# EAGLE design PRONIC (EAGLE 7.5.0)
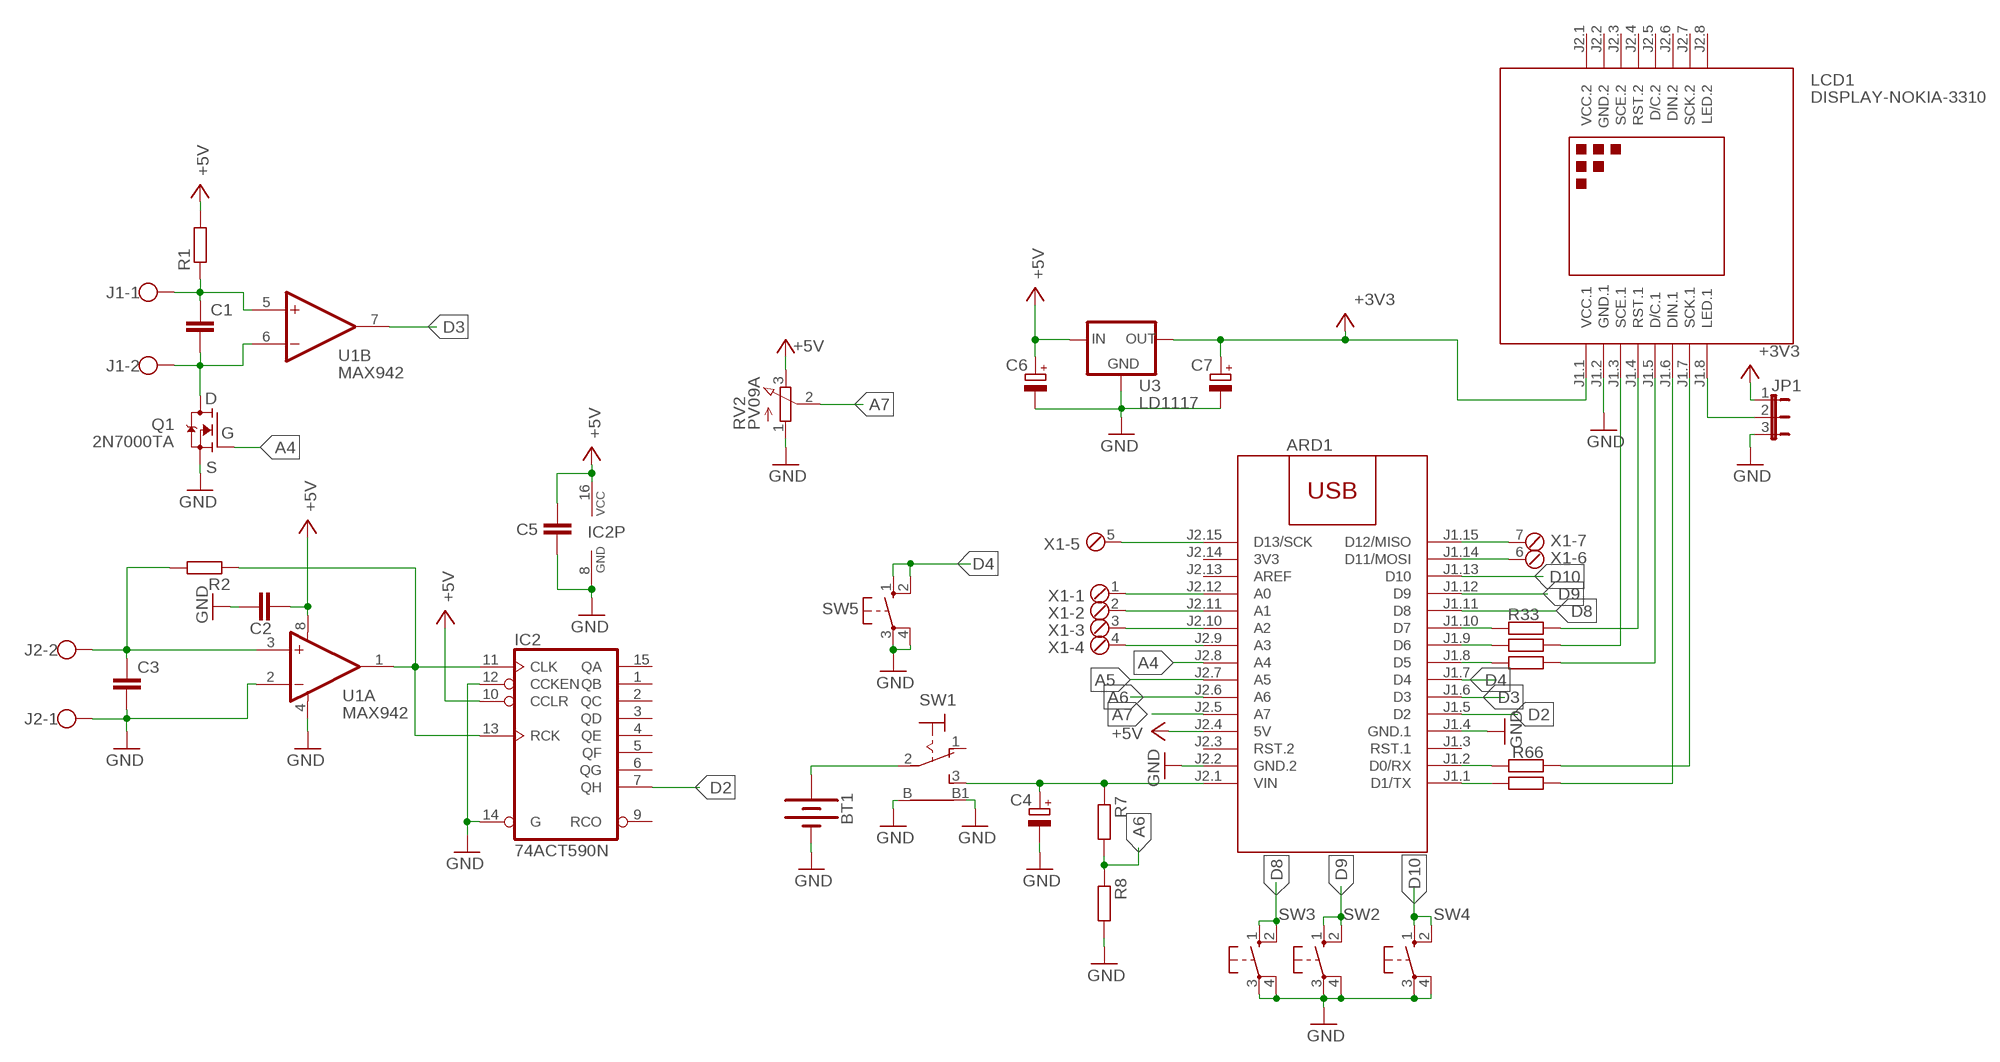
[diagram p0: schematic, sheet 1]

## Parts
ARD1  ARDUINO-NANO-3.0  [ARDUINO-NANO-3.0]
BT1  BATTERY-9V  [BATTCON_9V]
C1  C-EUC1206  [C1206]
C2  C-EUC1206  [C1206]
C3  C-EUC1206  [C1206]
C4  CPOL-EUSMCC  [SMC_C]
C5  C-EUC1206  [C1206]
C6  CPOL-EUSMCB  [SMC_B]
C7  CPOL-EUSMCB  [SMC_B]
IC2  74ACT590N  [DIL16]
J1  W237-102  [W237-102]
J2  W237-102  [W237-102]
JP1  JP2E  [JP2]
LCD1  DISPLAY-NOKIA-3310  [DISPLAY-NOKIA-3310]
Q1  2N7000TA  [TO-92]
R1  R-EU_R1206  [R1206]
R2  R-EU_R1206  [R1206]
R7  R-EU_R1206  [R1206]
R8  R-EU_R1206  [R1206]
R22  R-EU_R1206  [R1206]
R33  R-EU_R1206  [R1206]
R44  R-EU_R1206  [R1206]
R55  R-EU_R1206  [R1206]
R66  R-EU_R1206  [R1206]
RV2  PV09A  [PTV09]
SW1  9070-1W  [9070-1W]
SW2  40-XX  [B3F-40XX]
SW3  40-XX  [B3F-40XX]
SW4  40-XX  [B3F-40XX]
SW5  40-XX  [B3F-40XX]
U1  MAX942  MAX907CPA  [DIL08]
U3  LD1117  [SOT223]
X1  MPT7  [7POL254]

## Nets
+3V3: C7.+ JP1.1 LCD1.J1.1(VCC.1) U3.2(OUT)
+5V: ARD1.J2.4(5V) C2.2 C5.2 C6.+ IC2.10(CCLR) IC2.16(VCC) R1.2 RV2.3(E) U1.8(A:V+) U3.3(IN)
A4: ARD1.J2.8(A4) Q1.2(G)
A5: ARD1.J2.7(A5)
A6: ARD1.J2.6(A6) R7.2 R8.1
A7: ARD1.J2.5(A7) RV2.2(S)
D2: ARD1.J1.5(D2) IC2.7(QH)
D3: ARD1.J1.6(D3) U1.7(B:OUT)
D4: ARD1.J1.7(D4) SW5.1(S) SW5.2(S1)
D8: ARD1.J1.11(D8) SW3.1(S) SW3.2(S1)
D9: ARD1.J1.12(D9) SW2.1(S) SW2.2(S1)
D10: ARD1.J1.13(D10) SW4.1(S) SW4.2(S1)
GND: ARD1.J1.4(GND.1) ARD1.J2.2(GND.2) BT1.- C2.1 C3.2 C4.- C5.1 C6.- C7.- IC2.8(GND) IC2.12(CCKEN) IC2.14(G) J2.1 JP1.3 LCD1.J1.2(GND.1) Q1.1(S) R8.2 RV2.1(A) SW1.B SW1.B1 SW2.3(P) SW2.4(P1) SW3.3(P) SW3.4(P1) SW4.3(P) SW4.4(P1) SW5.3(P) SW5.4(P1) U1.2(A:-IN) U1.4(A:V-) U3.1(GND)
N$1: ARD1.J1.1(D1/TX) R55.2
N$2: LCD1.J1.6(DIN.1) R55.1
N$3: ARD1.J1.10(D7) R33.2
N$4: ARD1.J1.9(D6) R22.2
N$5: ARD1.J1.8(D5) R44.2
N$6: ARD1.J1.2(D0/RX) R66.2
N$7: ARD1.J2.12(A0) X1.1
N$8: LCD1.J1.4(RST.1) R33.1
N$9: LCD1.J1.3(SCE.1) R22.1
N$10: LCD1.J1.5(D/C.1) R44.1
N$11: ARD1.J2.11(A1) X1.2
N$12: LCD1.J1.7(SCK.1) R66.1
N$13: JP1.2 LCD1.J1.8(LED.1)
N$14: ARD1.J2.10(A2) X1.3
N$15: ARD1.J2.9(A3) X1.4
N$16: ARD1.J2.15(D13/SCK) X1.5
N$17: ARD1.J1.14(D11/MOSI) X1.6
N$18: ARD1.J1.15(D12/MISO) X1.7
N$19: C1.1 J1.1 R1.1 U1.5(B:+IN)
N$20: C1.2 J1.2 Q1.3(D) U1.6(B:-IN)
N$21: C3.1 J2.2 R2.2 U1.3(A:+IN)
N$22: IC2.11(CLK) IC2.13(RCK) R2.1 U1.1(A:OUT)
N$24: BT1.+ SW1.2(P)
N$25: ARD1.J2.1(VIN) C4.+ R7.1 SW1.3(S)
Unconnected: ARD1.J1.3(RST.1) ARD1.J2.3(RST.2) ARD1.J2.13(AREF) IC2.1(QB) IC2.2(QC) IC2.3(QD) IC2.4(QE) IC2.5(QF) IC2.6(QG) IC2.9(RCO) IC2.15(QA) LCD1.J2.3(SCE.2) LCD1.J2.4(RST.2) LCD1.J2.5(D/C.2) LCD1.J2.6(DIN.2) LCD1.J2.7(SCK.2) LCD1.J2.8(LED.2) SW1.1(O)

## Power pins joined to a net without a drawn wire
3V3: ARD1.J2.14(3V3)
GND.2: LCD1.J2.2(GND.2)
VCC.2: LCD1.J2.1(VCC.2)

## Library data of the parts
ARD1 = diy-modules:ARDUINO-NANO-3.0: Arduino Nano 3.0 and compatible devices More details available here: https://www.arduino.cc/en/Main/ArduinoBoardNano Click here to find device on ebay.com
BT1 = SparkFun-Batteries:BATTERY: Battery - Single Cell; PROD_ID: BATT-10855
C1-C3 C5 = rcl:C-EU: CAPACITOR, European symbol
C4 C6 C7 = rcl:CPOL-EU: POLARIZED CAPACITOR, European symbol
IC2 = 74xx-eu:74*590: 8-bit binary COUNTER, output register
J1 J2 = con-wago-500:W237-102: WAGO SCREW CLAMP; MPN: 237-102; OC_FARNELL: unknown; OC_NEWARK: 70K9898
JP1 = jumper:JP2E: JUMPER
LCD1 = diy-modules:DISPLAY-NOKIA-3310: 84x48 Dot Matrix LCD Module based on Nokia 3310 display More details available here: https://arduinoandsoftware.wordpress.com/2012/12/30/nokia-33105110-3-3v-display-with-5v-arduino/
Q1 = 2N7000TA:2N7000TA: http://www.mouser.com/ds/2/149/2N7000TA-347571.pdf Check availability; AVAILABILITY: In Stock; CHECK_PRICES: https://www.snapeda.com/parts/2N7000-TA/Onsemi/view-part/?ref=eda; DESCRIPTION: N-Channel 60 V 200mA (Tc) 400mW (Ta) Through Hole TO-92-3; MF: ON Semiconductor; MP: 2N7000-TA; PACKAGE: E-PKG AXIAL-LEADED-2 ON Semiconductor; PRICE: None; SNAPEDA_LINK: https://www.snapeda.com/parts/2N7000-TA/Onsemi/view-part/?ref=snap
R1 R2 R7 R8 R22 R33 R44 R55 R66 = rcl:R-EU_: RESISTOR, European symbol
RV2 = pot:PV09A
SW1 = switch:9070-1W: TOGGLE SWITCH Marquardt
SW2-SW5 = switch-omron:40-XX: OMRON SWITCH; MF: OMRON COMPONENTS USA; MPN: B3F-4000; OC_FARNELL: 176434; OC_NEWARK: 36K3105
U1 = maxim:MAX907CPA: COMPARATOR; MF: MAXIM; MPN: MAX907CPA; OC_FARNELL: unknown; OC_NEWARK: 79C3004
U3 = v-reg:LD1117
X1 = con-phoenix-254:MPT7: PHOENIX CONNECTOR; OC_FARNELL: unknown; OC_NEWARK: unknown

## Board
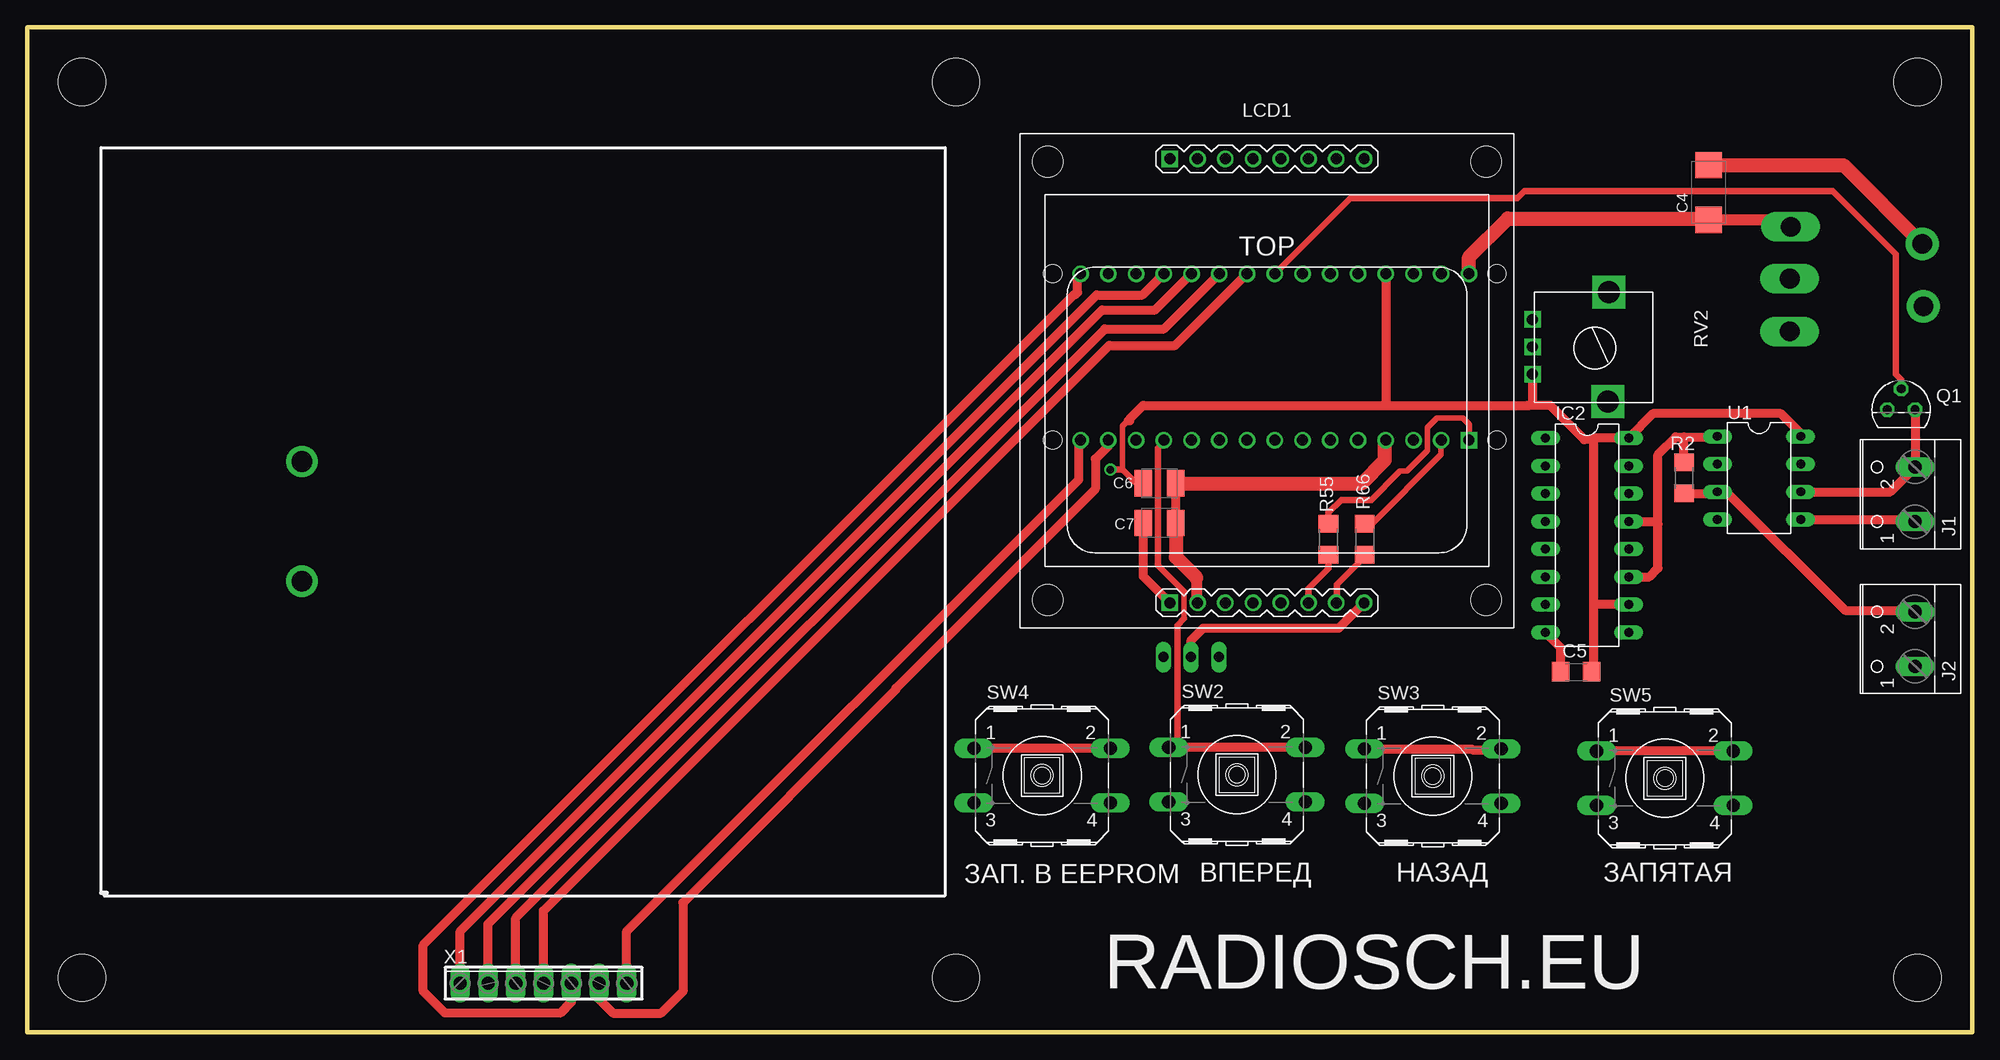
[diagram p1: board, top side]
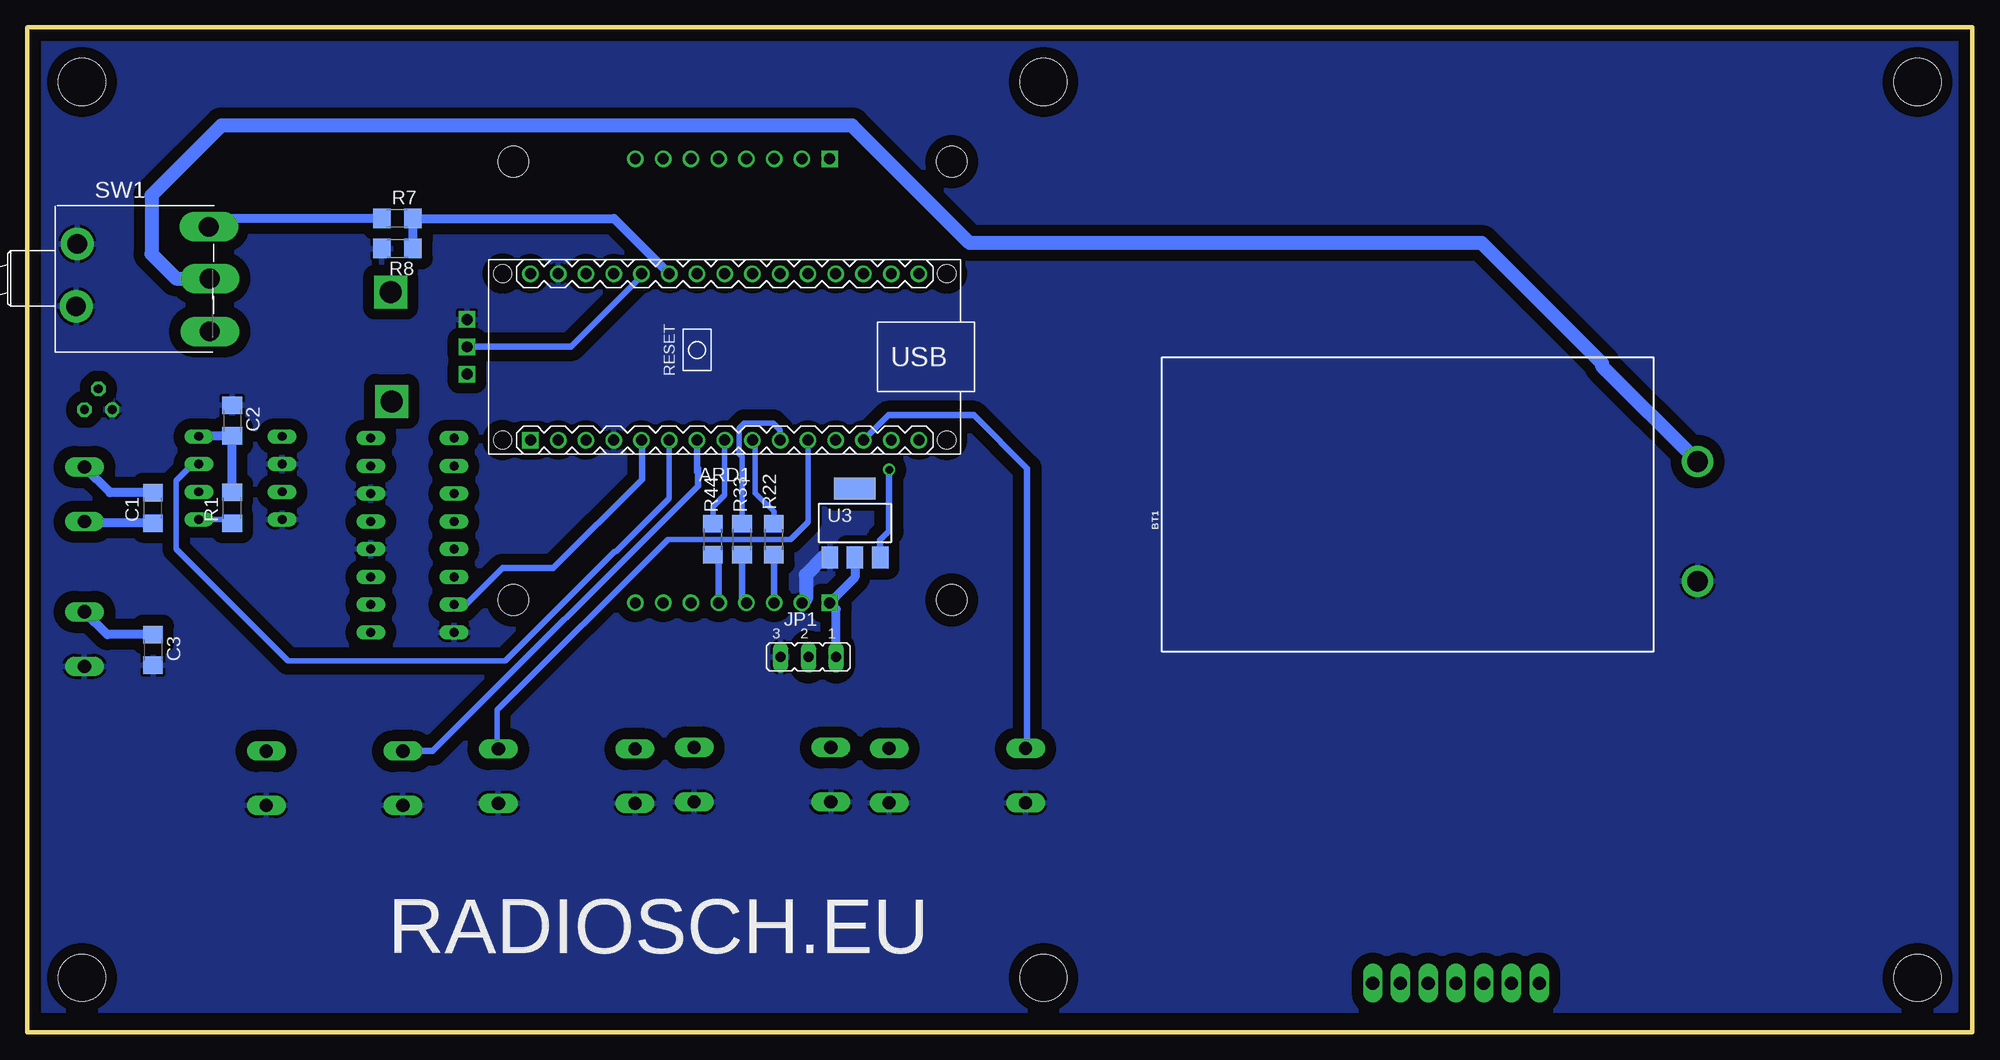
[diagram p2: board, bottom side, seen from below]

Size 178 x 92 mm. Coordinates in mm from the lower left corner, seen from the top.
Outline: 0,0 178,0 178,92 0,92 0,0
Copper layers (1*16): Top 0.035mm / dielectric 1.5mm / Bottom 0.035mm
Design rules "default": minimum track width 10mil, minimum drill 24mil, track to track 8mil, track to pad 8mil, pad to pad 8mil, via to via 8mil, smd to smd 8mil, copper to edge 40mil, drill to drill 8mil, minimum pad ring 10mil, minimum via ring 8mil, stop-mask expansion 4mil, vias tented up to drill 0mil, thermal gap 10mil
Holes 4.3 mm at 5,5 173,5 5,87 85,5 85,87 173,87

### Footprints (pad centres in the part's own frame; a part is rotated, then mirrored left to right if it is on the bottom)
ARDUINO-NANO-3.0 = drill 1 square: J1.1 17.78,7.62 | drill 1: J1.2 15.24,7.62; J1.3 12.7,7.62; J1.4 10.16,7.62; J1.5 7.62,7.62; J1.6 5.08,7.62; J1.7 2.54,7.62; J1.8 0,7.62; J1.9 -2.54,7.62; J1.10 -5.08,7.62; J1.11 -7.62,7.62; J1.12 -10.16,7.62; J1.13 -12.7,7.62; J1.14 -15.24,7.62; J1.15 -17.78,7.62; J2.1 17.78,-7.62; J2.2 15.24,-7.62; J2.3 12.7,-7.62; J2.4 10.16,-7.62; J2.5 7.62,-7.62; J2.6 5.08,-7.62; J2.7 2.54,-7.62; J2.8 0,-7.62; J2.9 -2.54,-7.62; J2.10 -5.08,-7.62; J2.11 -7.62,-7.62; J2.12 -10.16,-7.62; J2.13 -12.7,-7.62; J2.14 -15.24,-7.62; J2.15 -17.78,-7.62 | hole 1.651: -20.32,7.62; -20.32,-7.62; 20.32,-7.62; 20.32,7.62
BATTCON_9V = drill 1.905: + -4,-1; - -4,-11.954
C1206 = smd 1.6 x 1.8: 1 -1.4,0; 2 1.4,0
SMC_C = smd 2.4 x 2.4: + -2.5,0; - 2.5,0
SMC_B = smd 1.6 x 2.4: + -1.5,0; - 1.5,0
DIL16 = drill 0.813 long: 1 -8.89,-3.81; 2 -6.35,-3.81; 3 -3.81,-3.81; 4 -1.27,-3.81; 5 1.27,-3.81; 6 3.81,-3.81; 7 6.35,-3.81; 8 8.89,-3.81; 9 8.89,3.81; 10 6.35,3.81; 11 3.81,3.81; 12 1.27,3.81; 13 -1.27,3.81; 14 -3.81,3.81; 15 -6.35,3.81; 16 -8.89,3.81
W237-102 = drill 1.194 long: 1 -2.5,-1.27; 2 2.5,-1.27
JP2 = drill 0.914 long: 1 -2.54,0; 2 0,0; 3 2.54,0
DISPLAY-NOKIA-3310 = drill 1 square: J1.1 -8.89,-20.32; J2.1 -8.89,20.32 | drill 1: J1.2 -6.35,-20.32; J1.3 -3.81,-20.32; J1.4 -1.27,-20.32; J1.5 1.27,-20.32; J1.6 3.81,-20.32; J1.7 6.35,-20.32; J1.8 8.89,-20.32; J2.2 -6.35,20.32; J2.3 -3.81,20.32; J2.4 -1.27,20.32; J2.5 1.27,20.32; J2.6 3.81,20.32; J2.7 6.35,20.32; J2.8 8.89,20.32 | hole 2.8: -20.066,-20.066; 20.066,-20.066; 20.066,20.066; -20.066,20.066
TO-92 = drill 0.813 octagon: 1 -1.27,0; 2 0,1.905; 3 1.27,0
R1206 = smd 1.6 x 1.803: 1 -1.422,0; 2 1.422,0
PTV09 = drill 1 square: 1 -2.5,0; 2 0,0; 3 2.5,0 | drill 2 square: P$4 -5,7; P$5 5,6.9
9070-1W = drill 1.813 long: 1 5.08,-4.835; 2 5.08,0 | drill 1.8 long: 3 4.98,4.735 | drill 1.8 pad 3: B -7.161,-2.544; B1 -7.061,3.167
B3F-40XX = drill 1.194 long: 1 -6.248,2.489; 2 6.248,2.489; 3 -6.248,-2.489; 4 6.248,-2.489
DIL08 = drill 0.813 long: 1 -3.81,-3.81; 2 -1.27,-3.81; 3 1.27,-3.81; 4 3.81,-3.81; 5 3.81,3.81; 6 1.27,3.81; 7 -1.27,3.81; 8 -3.81,3.81
SOT223 = smd 1.5 x 2: 1 -2.3,-3.15; 2 0,-3.15; 3 2.3,-3.15 | smd 3.8 x 2: 4 0,3.15
7POL254 = drill 1.2 long: 1 -7.62,0; 2 -5.08,0; 3 -2.54,0; 4 0,0; 5 2.54,0; 6 5.08,0; 7 7.62,0

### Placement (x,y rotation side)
ARD1  114.17,61.83 180 bottom
BT1  21.12,53.25 0 bottom
C1  166.5,48 90 bottom
C2  159.25,56 270 bottom
C3  166.5,35 270 bottom
C4  153.88,76.88 90 top
C5  141.75,33 0 top
C6  103.62,50.25 0 top
C7  103.62,46.62 0 top
IC2  142.75,45.5 270 top
J1  171.5,49.25 90 top
J2  171.5,36 90 top
JP1  106.51,34.35 180 bottom
LCD1  113.46,59.64 0 top
Q1  171.5,57 0 top
R1  159.25,48 90 bottom
R2  151.62,50.75 270 top
R7  144.12,74.5 0 bottom
R8  144.12,71.75 180 bottom
R22  109.67,45.13 90 bottom
R33  112.59,45.13 90 bottom
R44  115.25,45.13 90 bottom
R55  119.08,45.13 90 top
R66  122.41,45.13 90 top
RV2  137.75,62.75 270 top
SW1  166.38,69 0 bottom
SW2  110.71,23.58 0 top
SW3  128.64,23.45 0 top
SW4  92.88,23.5 0 top
SW5  149.88,23.25 0 top
U1  158.5,50.75 270 top
U3  102.25,46.62 0 bottom
X1  47.25,4.5 0 top

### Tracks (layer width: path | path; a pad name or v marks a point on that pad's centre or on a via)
+3V3
  Top 0.813: C7.+ 102.12,41.77 LCD1.J1.1
  Bottom 0.813: JP1.1 103.97,38.72 LCD1.J1.1 102.25,41.64 U3.2
+5V  (via drill 0.7)
  Top 0.5: C6.+ 101.5,50.25 100.25,51.5 100.25,55.5 100.75,56
  Top 0.61: v99.12,51.5 100.25,51.5
  Top 0.813: 100.75,56 100.88,56 100.88,56.12 102.12,57.38 124.62,57.38 | 124.62,57.38 137.25,57.38 137.5,57.38 | 143.38,39 143.38,33.23 C5.2 | 143.38,39 143.38,54.25 | 143.38,54.25 143.51,54.39 IC2.16 148.79,56.62 160.5,56.62 162.31,54.81 U1.8 | ARD1.J2.4 124.33,57.67 124.62,57.38 | IC2.10 143.53,39.15 143.38,39 | RV2.3 137.75,57.62 137.5,57.38 | 143.38,54.25 142.5,54.25 139.38,57.38 137.5,57.38
  Bottom 0.61: U3.3 99.95,45.05 99.12,45.88 v99.12,51.5
  Bottom 0.813: R1.2 C2.2 162.27,54.6 U1.8
A4
  Top 0.61: ARD1.J2.8 121.09,76.38 136.38,76.38 137,77 165.25,77 171,71.25 171,60.25 171.5,59.75 Q1.2
A6
  Bottom 0.813: ARD1.J2.6 124.3,74.5 R7.2 R8.1
A7
  Bottom 0.61: RV2.2 128.25,62.75 122.12,68.88 122.12,69.11 ARD1.J2.5
D2
  Bottom 0.61: IC2.7 137.85,39.15 134.5,42.5 129.88,42.5 121.75,50.62 121.75,54.17 ARD1.J1.5
D3
  Bottom 0.5: ARD1.J1.6 119.25,48.88 124.12,44 124.25,44 134.25,34 154.12,34 164.38,44.25 164.38,50.5 162.88,52 162.33,52 U1.7
D4
  Top 0.813: SW5.2 SW5.1
  Bottom 0.61: ARD1.J1.7 116.71,51.75 | 116.71,51.75 116.71,51.29 | SW5.1 140.89,25.74 116.62,50 116.62,51.66 116.71,51.75
D8
  Top 0.813: 122.41,25.95 SW3.1 132.19,25.94 132.25,25.88 134.82,25.88 SW3.2
  Bottom 0.5: ARD1.J1.11 106.55,46.7 108.12,45.12 119.38,45.12 135,29.5 135,26.05 SW3.2
D9
  Top 0.5: 105.88,40.38 105.88,37.88
  Top 0.61: ARD1.J1.12 104.01,54.01 103.5,53.5 103.5,42.75 105.88,40.38 | 105.88,37.88 105.25,37.25 105.25,26.86 SW2.1
  Top 0.813: SW2.2 SW2.1
D10
  Top 0.813: SW4.2 SW4.1
  Bottom 0.61: SW4.1 86.5,26.12 86.5,51.62 91.38,56.5 99.18,56.5 ARD1.J1.13
GND
  Top 0.813: C7.- C6.- | C5.1 140.35,35.2 IC2.8
  Top 1.016: 107,41.62 107,39.43
  Top 1.27: C6.- 122.12,50.25 124.25,52.38 124.25,54.13 ARD1.J1.4 | C7.- 105.12,43.5 107,41.62 | 107,39.43 LCD1.J1.2 | C4.- 166.23,79.38 SW1.B1
  Bottom 1.27: U3.1 105.15,43.48 106.75,41.88 106.75,39.68 LCD1.J1.2
  pour Bottom (isolate 1.016): 1.5,2 177,2 177,91 1.5,91
N$1
  Top 0.5: 125.5,51.25 125.62,51.38 126.25,51.38 128.12,53.25 128.12,55.38 129,56.25 131.38,56.25 132,55.62 132,54.26 ARD1.J1.1
  Top 0.61: R55.2 119.08,47.58 120.25,48.75 123,48.75 125.5,51.25
N$2
  Top 0.61: R55.1 119.08,42.45 117.25,40.62 117.25,39.34 LCD1.J1.6
N$3
  Bottom 0.5: R33.2 112.59,52.72 112.88,53 112.88,55.25 112.38,55.75 109.75,55.75 109.12,55.12 109.12,54.24 ARD1.J1.10
N$4
  Bottom 0.5: R22.2 109.67,47.67 111.38,49.38 111.38,53.95 ARD1.J1.9
N$5
  Bottom 0.5: ARD1.J1.8 114.17,49.2 115.25,48.12 R44.2
N$6
  Top 0.5: R66.2 123.05,46.55 129.38,52.88 129.38,54.17 ARD1.J1.2
N$7
  Top 0.813: X1.1 39.63,9.26 97.88,67.5 102.06,67.5 ARD1.J2.12
N$8
  Bottom 0.61: R33.1 112.59,39.72 LCD1.J1.4
N$9
  Bottom 0.61: R22.1 109.67,39.34 LCD1.J1.3
N$10
  Bottom 0.61: LCD1.J1.5 114.73,43.19 R44.1
N$11
  Top 0.813: X1.2 42.17,9.92 98.38,66.12 103.22,66.12 ARD1.J2.11
N$12
  Top 0.61: R66.1 122.41,43.53 119.88,41 119.88,39.38 LCD1.J1.7
N$13
  Top 0.813: JP1.2 106.51,35.88 107.62,37 120.03,37 LCD1.J1.8
N$14
  Top 0.813: X1.3 44.71,10.46 98.62,64.38 104.02,64.38 ARD1.J2.10
N$15
  Top 0.813: X1.4 47.25,11.12 99,62.88 105.06,62.88 ARD1.J2.9
N$16
  Top 0.813: X1.5 49.79,2.79 48.75,1.75 38.25,1.75 36.25,3.75 36.25,8 95.75,67.5 95.88,67.5 96.12,67.75 96.12,69.19 ARD1.J2.15
N$17
  Top 0.813: ARD1.J1.14 98.93,53.68 97.75,52.5 97.75,49.75 79.5,31.5 79.5,31.38 60,11.88 60,3.75 58,1.75 53.62,1.75 52.25,3.12 52.25,4.42 X1.6
N$18
  Top 0.813: X1.7 54.87,9.24 96.25,50.62 96.25,54.07 ARD1.J1.15
N$19
  Top 0.813: U1.5 172.58,46.94 J1.1
  Bottom 0.5: U1.5 159.61,46.94 R1.1
  Bottom 0.813: C1.1 172.62,46.6 J1.1
N$20
  Top 0.813: U1.6 170.5,49.48 J1.2 Q1.3
  Bottom 0.813: C1.2 170.42,49.4 J1.2
N$21
  Top 0.813: R2.2 154.54,49.33 U1.3 155.52,49.48 166.38,38.62 172.65,38.62 J2.2
  Bottom 0.813: C3.1 170.67,36.4 J2.2
N$22
  Top 0.813: IC2.11 148.44,41.69 149.25,42.5 149.25,46.5 | 149.25,46.5 149.25,52.88 150.88,54.5 151.62,54.5 | 151.62,54.5 154.63,54.5 U1.1 | R2.1 151.62,54.5 | IC2.13 148.98,46.77 149.25,46.5
N$24
  Bottom 1.27: BT1.+ 33.88,61 33.88,61.25 44.88,72.25 91.75,72.25 102.5,83 160.25,83 166.62,76.62 166.62,71.25 164.38,69 162,69 161.88,69.12 161.42,69.12 SW1.2
N$25
  Top 1.016: C4.+ 160.75,74.38 SW1.3
  Top 1.27: ARD1.J2.1 131.95,70.95 135.5,74.5 153.75,74.5 C4.+
  Bottom 0.813: R7.1 160.63,74.5 SW1.3

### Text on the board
tPlace: ЗАП. В EEPROM | ВПЕРЕД | НАЗАД | ЗАПЯТАЯ | RADIOSCH.EU
bPlace: RADIOSCH.EU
